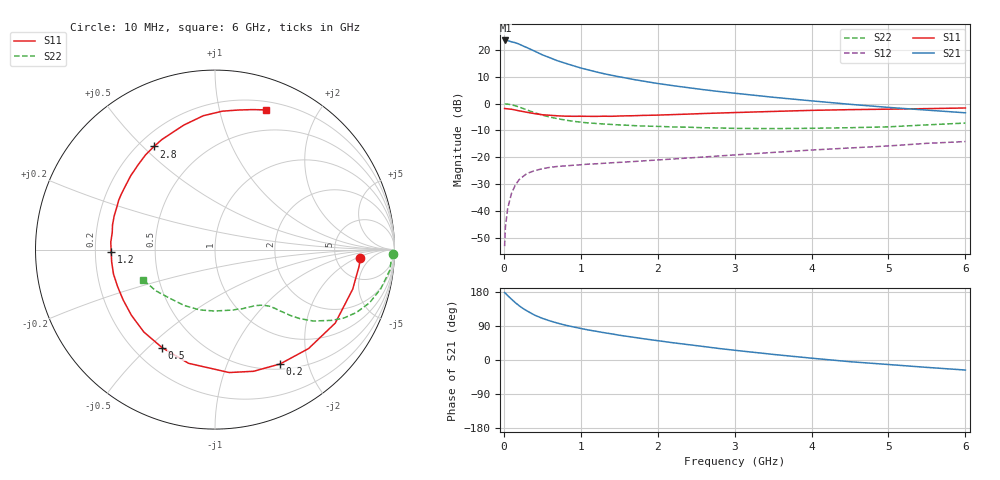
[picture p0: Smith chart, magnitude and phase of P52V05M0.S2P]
! SIEMENS Small Signal Semiconductors
! BFP183
! Si NPN RF Bipolar Junction Transistor in SOT143
! VCE = 2 V  IC = 5 mA
! Common Emitter S-Parameters:  March  1996
# GHz  S  MA  R  50
!  f  S11  S21  S12  S22
! GHz  MAG  ANG  MAG  ANG  MAG  ANG  MAG  ANG
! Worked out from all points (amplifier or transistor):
!   36 points, 10 MHz to 6 GHz, reference 50 ohm
!   highest |S21| = 23.6 dB at 20 MHz (marker M1)
!   |S21| within 3 dB of that: start of sweep to 325.6 MHz
!   unconditionally stable (mu >= 1): 1.539 GHz to 5.674 GHz
!   at 250 MHz: K = 0.21, MSG = 24.3 dB, |S12| = -27.2 dB
!   at 1.4 GHz: K = 0.95, MSG = 16.3 dB, |S12| = -22.1 dB
!   at 6 GHz: K = 0.95, MSG = 5.4 dB, |S12| = -14.1 dB
!   lowest NFmin = 1.15 dB at 450 MHz
!   S11 on the Smith chart (normalised r, x): 10 MHz: 8.91, -2.43; 200 MHz: 0.57, -1.57; 500 MHz: 0.31, -0.55; 1.2 GHz: 0.27, -0.01; 2.8 GHz: 0.26, +0.54; 6 GHz: 0.28, +1.40
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0.01  0.811 -3.3  14.89 178.1  0.0022 84.8  0.9929 -1.4
0.02  0.8079 -6.7  15.05 176.4  0.0049 88.2  0.985 -2.7
0.05  0.7983 -16.0  14.93 170.0  0.0112 82.8  0.9807 -6.7
0.1  0.7852 -31.4  14.2 160.4  0.0213 73.3  0.9495 -13.2
0.15  0.7588 -46.6  13.65 151.2  0.0305 67.1  0.9107 -19.0
0.2  0.7332 -60.3  12.85 143.1  0.0384 60.7  0.8621 -24.0
0.25  0.7112 -72.4  11.87 135.8  0.0439 55.1  0.8126 -28.0
0.3  0.6895 -83.4  11.08 129.7  0.0498 51.1  0.7629 -31.1
0.4  0.6505 -103.1  9.511 118.4  0.0563 43.8  0.677 -36.0
0.5  0.6206 -118.3  8.134 110.0  0.0611 38.8  0.61 -39.1
0.6  0.6066 -130.8  7.153 103.1  0.065 35.7  0.5619 -41.0
0.7  0.5923 -141.8  6.278 97.2  0.0675 33.6  0.5226 -42.3
0.8  0.5836 -151.1  5.653 91.9  0.069 31.8  0.4934 -43.5
1.1  0.5798 -173.1  4.247 79.2  0.0745 29.7  0.4365 -46.2
1.2  0.5786 -178.8  3.905 75.8  0.0755 29.1  0.427 -47.2
1.7  0.5955 157.0  2.799 59.6  0.0835 30.2  0.3883 -53.4
2.2  0.6245 138.7  2.161 45.5  0.0928 30.9  0.3679 -61.3
2.8  0.6678 120.6  1.68 30.3  0.1058 31.0  0.3514 -73.4
3.5  0.7151 104.1  1.315 14.8  0.123 30.1  0.3423 -90.4
4.5  0.7722 87.0  0.971 -4.5  0.149 26.0  0.3555 -119.0
5.5  0.8071 75.1  0.757 -19.5  0.1818 21.0  0.4016 -145.1
6  0.8294 69.8  0.674 -26.5  0.1963 17.1  0.4339 -157.1
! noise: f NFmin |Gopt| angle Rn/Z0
0.45  1.15  0.25  40  0.26
0.9  1.2  0.25  93  0.22
1.8  1.95  0.32  170  0.13
